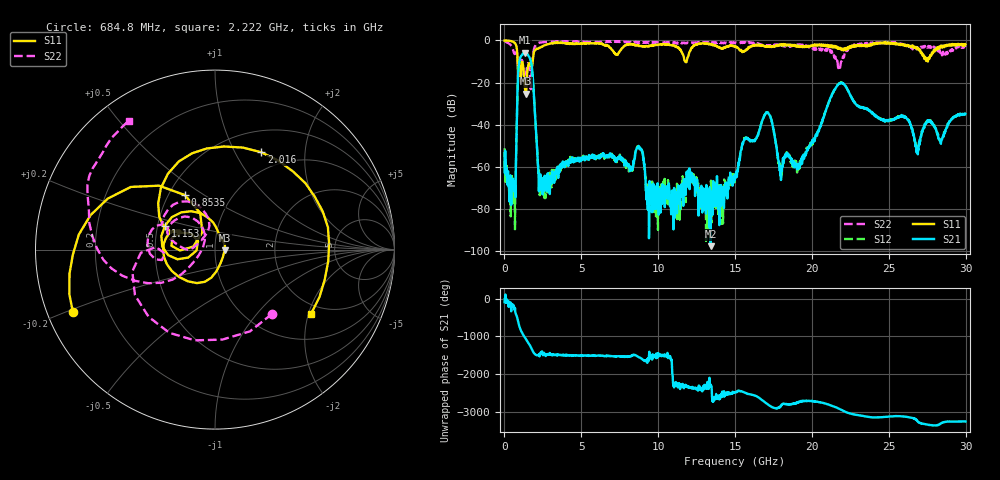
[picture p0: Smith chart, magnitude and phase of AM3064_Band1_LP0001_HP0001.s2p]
# Hz S DB R 50.0
!freq dBS11 angS11 dBS21 angS21 dBS12 angS12 dBS22 angS22
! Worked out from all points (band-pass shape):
!   1600 points, 10 MHz to 29.98 GHz, reference 50 ohm
!   highest |S21| = -5.81 dB at 1.322 GHz (marker M1); lowest = -97.7 dB at 13.41 GHz (marker M2)
!   |S21| within 3 dB of the highest: 1.004 GHz to 1.676 GHz (671.5 MHz wide, 50.1 % of centre)
!   lowest |S11| = -25.4 dB at 1.397 GHz (marker M3), VSWR 1.11, Z = 55.7 - j0.479 ohm
!   |S11| at or under -10 dB: 857.3 MHz to 1.829 GHz (971.9 MHz wide, 72.4 % of centre); 11.75 GHz to 11.84 GHz (98.14 MHz wide, 0.832 % of centre); 27.54392 GHz to 27.54461 GHz (692 kHz wide, 0.00251 % of centre)
!   |S22| runs from -23.2 to -0.2 dB; largest |S21 - S12| = 0.0054
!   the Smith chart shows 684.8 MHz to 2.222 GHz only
!   S11 on the Smith chart (normalised r, x): 684.8 MHz: 0.08, -0.21; 853.5 MHz: 0.60, +0.42; 1.153 GHz: 0.55, +0.16; 2.016 GHz: 0.76, +1.29; 2.222 GHz: 1.71, -2.08
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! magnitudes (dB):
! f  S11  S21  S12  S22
! 10 MHz  0.0  -53.6  -51.2  -0.2
! 684.8 MHz  -1.3  -68.6  -89.7  -6.4
! 853.5 MHz  -9.2  -22.7  -22.6  -9.6
! 1.153 GHz  -10.2  -6.9  -6.8  -9.6
! 1.322 GHz  -22.3  -5.8  -5.8  -20.7
! 1.397 GHz  -25.4  -5.9  -5.9  -16.2
! 1.734 GHz  -12.8  -10.4  -10.4  -20.2
! 2.016 GHz  -4.4  -38.6  -38.5  -2.4
! 2.222 GHz  -3.8  -64.2  -63.2  -1.3
! 5.015 GHz  -1.4  -56.2  -56.7  -0.6
! 8.763 GHz  -2.7  -50.7  -50.9  -1.1
! 9.344 GHz  -2.8  -69.8  -80.4  -0.9
! 10 GHz  -2.0  -70.0  -74.7  -0.9
! 13.41 GHz  -2.0  -97.7  -69.7  -1.2
! 15 GHz  -3.0  -63.9  -65.5  -1.2
! 17.05 GHz  -2.9  -34.4  -34.2  -2.8
! 17.97 GHz  -2.3  -62.4  -61.3  -2.1
! 19.99 GHz  -2.8  -48.8  -48.4  -3.3
! 21.87 GHz  -3.8  -20.2  -20.3  -11.3
! 25 GHz  -1.0  -37.8  -38.1  -1.1
! 26.85 GHz  -4.3  -53.6  -51.5  -3.2
! 29.98 GHz  -1.9  -34.9  -34.8  -3.2
